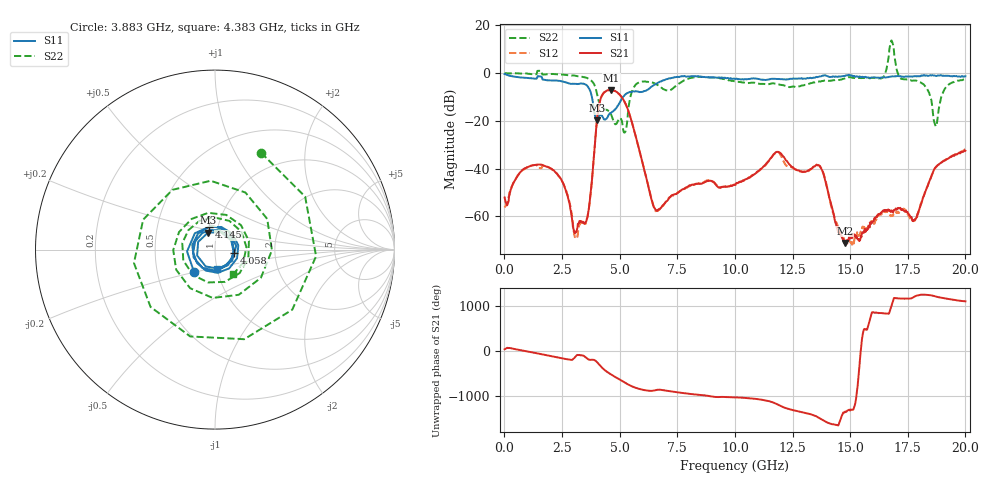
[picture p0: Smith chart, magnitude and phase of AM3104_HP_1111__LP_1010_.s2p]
!Created with skrf (http://scikit-rf.org).
# Hz S RI R 50.0
!freq ReS11 ImS11 ReS21 ImS21 ReS12 ImS12 ReS22 ImS22
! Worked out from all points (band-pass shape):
!   1601 points, 10 MHz to 20 GHz, reference 50 ohm
!   highest |S21| = -7.06 dB at 4.633 GHz (marker M1); lowest = -71.2 dB at 14.77 GHz (marker M2)
!   |S21| within 3 dB of the highest: 4.2 GHz to 5.089 GHz (888.2 MHz wide, 19.1 % of centre)
!   lowest |S11| = -19.8 dB at 4.02 GHz (marker M3), VSWR 1.23, Z = 45.3 + j8.61 ohm
!   |S11| at or under -10 dB: 3.797 GHz to 5.15 GHz (1.353 GHz wide, 30.2 % of centre)
!   |S22| runs from -25.0 to 13.7 dB; largest |S21 - S12| = 0.032
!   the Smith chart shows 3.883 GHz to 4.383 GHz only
!   S11 on the Smith chart (normalised r, x): 3.883 GHz: 0.77, -0.19; 4.058 GHz: 1.23, -0.05; 4.145 GHz: 0.90, +0.23; 4.383 GHz: 1.01, -0.21
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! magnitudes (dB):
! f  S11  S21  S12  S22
! 10 MHz  -0.4  -52.1  -56.3  0.0
! 1.759 GHz  -2.9  -38.9  -39.0  -0.6
! 3.083 GHz  -4.5  -66.5  -68.6  -1.1
! 3.346 GHz  -4.4  -62.1  -62.5  -1.5
! 3.621 GHz  -5.7  -59.2  -59.3  -2.2
! 3.883 GHz  -15.4  -35.1  -35.1  -4.5
! 4.02 GHz  -19.8  -19.5  -19.5  -8.9
! 4.058 GHz  -19.4  -16.5  -16.5  -10.5
! 4.145 GHz  -17.7  -11.8  -11.8  -13.4
! 4.383 GHz  -19.4  -7.8  -7.8  -15.3
! 4.633 GHz  -16.6  -7.1  -7.2  -17.4
! 5.32 GHz  -8.4  -14.3  -14.3  -21.1
! 5.707 GHz  -7.6  -26.9  -26.9  -4.7
! 6.682 GHz  -4.0  -57.2  -57.5  -5.1
! 10.01 GHz  -2.5  -46.8  -46.9  -3.5
! 11.82 GHz  -2.5  -33.0  -33.1  -4.6
! 13.34 GHz  -2.1  -40.0  -40.0  -4.2
! 14.77 GHz  -1.2  -71.2  -70.2  -2.2
! 16.68 GHz  -1.6  -57.5  -59.0  7.3
! 17.8 GHz  -1.3  -61.4  -61.8  -3.1
! 18.7 GHz  -1.2  -39.6  -39.6  -22.0
! 20 GHz  -1.4  -32.6  -31.9  -2.6
